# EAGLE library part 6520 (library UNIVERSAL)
pic18f6520 PUZDRO TQFP64 na redukcii
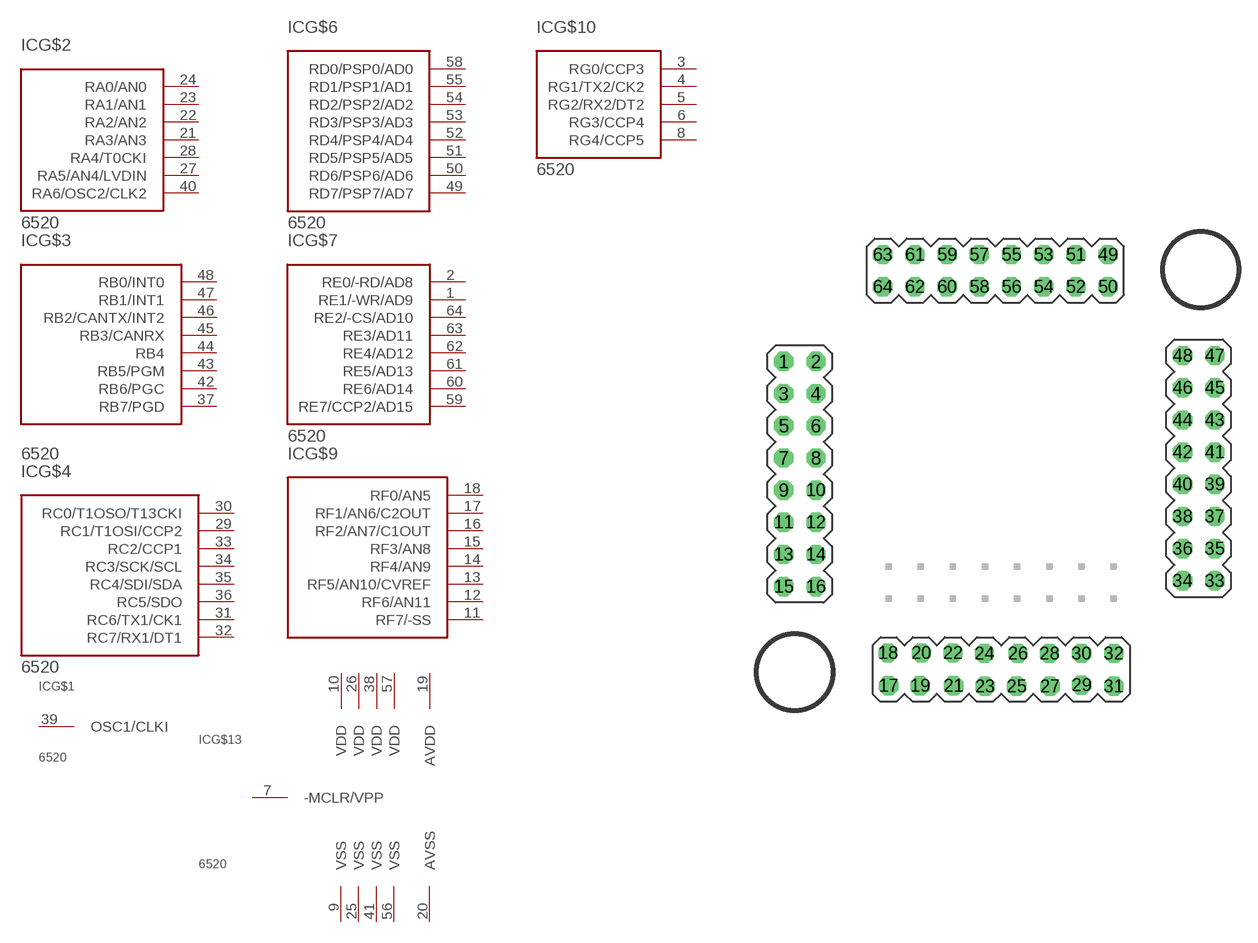
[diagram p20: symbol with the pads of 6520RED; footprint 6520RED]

Designator prefix IC; gates G$1=6520OSC G$2=6520PA G$3=6520PB G$4=6520PC G$6=6520PD G$7=6520PE G$9=6520PF G$10=6520PG G$13=6520PW

## 6520  [6520RED]
1  G$7:RE1/-WR/AD9
2  G$7:RE0/-RD/AD8
3  G$10:RG0/CCP3
4  G$10:RG1/TX2/CK2
5  G$10:RG2/RX2/DT2
6  G$10:RG3/CCP4
7  G$13:-MCLR/VPP  in
8  G$10:RG4/CCP5
9  G$13:VSS  pwr
10  G$13:VDD  pwr
11  G$9:RF7/-SS
12  G$9:RF6/AN11
13  G$9:RF5/AN10/CVREF
14  G$9:RF4/AN9
15  G$9:RF3/AN8
16  G$9:RF2/AN7/C1OUT
17  G$9:RF1/AN6/C2OUT
18  G$9:RF0/AN5
19  G$13:AVDD  pwr
20  G$13:AVSS  pwr
21  G$2:RA3/AN3
22  G$2:RA2/AN2
23  G$2:RA1/AN1
24  G$2:RA0/AN0
25  G$13:VSS  pwr
26  G$13:VDD  pwr
27  G$2:RA5/AN4/LVDIN
28  G$2:RA4/T0CKI
29  G$4:RC1/T1OSI/CCP2
30  G$4:RC0/T1OSO/T13CKI
31  G$4:RC6/TX1/CK1
32  G$4:RC7/RX1/DT1
33  G$4:RC2/CCP1
34  G$4:RC3/SCK/SCL
35  G$4:RC4/SDI/SDA
36  G$4:RC5/SDO
37  G$3:RB7/PGD
38  G$13:VDD  pwr
39  G$1:OSC1/CLKI  in
40  G$2:RA6/OSC2/CLK2
41  G$13:VSS  pwr
42  G$3:RB6/PGC
43  G$3:RB5/PGM
44  G$3:RB4
45  G$3:RB3/CANRX
46  G$3:RB2/CANTX/INT2
47  G$3:RB1/INT1
48  G$3:RB0/INT0
49  G$6:RD7/PSP7/AD7
50  G$6:RD6/PSP6/AD6
51  G$6:RD5/PSP5/AD5
52  G$6:RD4/PSP4/AD4
53  G$6:RD3/PSP3/AD3
54  G$6:RD2/PSP2/AD2
55  G$6:RD1/PSP1/AD1
56  G$13:VSS  pwr
57  G$13:VDD  pwr
58  G$6:RD0/PSP0/AD0
59  G$7:RE7/CCP2/AD15
60  G$7:RE6/AD14
61  G$7:RE5/AD13
62  G$7:RE4/AD12
63  G$7:RE3/AD11
64  G$7:RE2/-CS/AD10

## Footprint 6520RED (pad centres in mm)
drill 1.016 octagon: 1 -15.494,10.566; 2 -12.954,10.566; 3 -15.494,8.026; 4 -12.954,8.026; 5 -15.494,5.486; 6 -12.954,5.486; 7 -15.494,2.946; 8 -12.954,2.946; 9 -15.494,0.406; 10 -12.954,0.406; 11 -15.494,-2.134; 12 -12.954,-2.134; 13 -15.494,-4.674; 14 -12.954,-4.674; 15 -15.494,-7.214; 16 -12.954,-7.214; 17 -7.214,-15.037; 18 -7.264,-12.446; 19 -4.724,-15.037; 20 -4.623,-12.446; 21 -2.083,-15.037; 22 -2.134,-12.446; 23 0.406,-15.088; 24 0.356,-12.497; 25 2.896,-15.088; 26 2.997,-12.497; 27 5.537,-15.088; 28 5.486,-12.497; 29 8.026,-14.986; 30 8.026,-12.497; 31 10.566,-15.088; 32 10.566,-12.497; 33 18.542,-6.756; 34 16.002,-6.756; 35 18.542,-4.216; 36 16.002,-4.216; 37 18.542,-1.676; 38 16.002,-1.676; 39 18.542,0.864; 40 16.002,0.864; 41 18.542,3.404; 42 16.002,3.404; 43 18.542,5.944; 44 16.002,5.944; 45 18.542,8.484; 46 16.002,8.484; 47 18.542,11.024; 48 16.002,11.024; 49 10.109,18.999; 50 10.109,16.459; 51 7.569,18.999; 52 7.569,16.459; 53 5.029,18.999; 54 5.029,16.459; 55 2.489,18.999; 56 2.489,16.459; 57 -0.051,18.999; 58 -0.051,16.459; 59 -2.591,18.999; 60 -2.591,16.459; 61 -5.131,18.999; 62 -5.131,16.459; 63 -7.671,18.999; 64 -7.671,16.459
